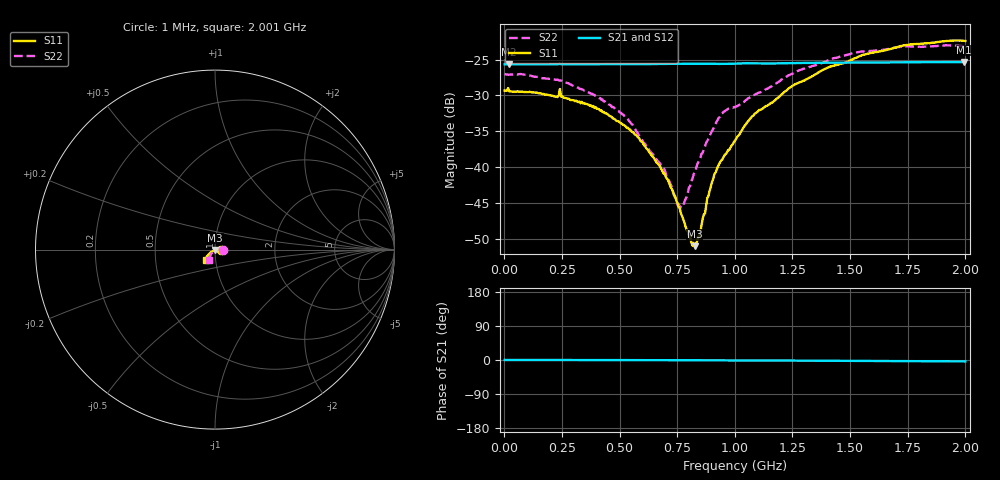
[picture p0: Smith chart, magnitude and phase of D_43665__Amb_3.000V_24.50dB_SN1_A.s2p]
! device id: 43665_
! dir: \\malibu\benchdata\1_engineers\tn_data\43665_75ohm\new\sparar\43665_\amb\3p000v\24p50db
! Serial: 1
! Insertion: A
! Temp: Amb
! VDD: 3.000V
! Attenuation Step: 24.50dB
! IDD: 1.450665e+00mA
! FILE NAME
! DATE 03-27-2009 08:39:23
! CORRECTED  DATA
#  Hz  S  RI  R  75
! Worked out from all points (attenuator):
!   401 points, 1 MHz to 2.001 GHz, reference 75 ohm
!   highest |S21| = -25.32 dB at 1.996 GHz (marker M1); lowest = -25.7 dB at 21 MHz (marker M2)
!   lowest |S11| = -51.0 dB at 826 MHz (marker M3), VSWR 1.01, Z = 75.1 - j0.413 ohm
!   |S11| at or under -10 dB: start of sweep to end of sweep
!   |S22| runs from -45.6 to -23.0 dB; largest |S21 - S12| = 0.00057
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1000000  0.0342 -0.000123  0.0522 3.89e-05  0.0521 -2.09e-05  0.0447 -0.000493
2.1e7  0.0338 0.000184  0.0521 -9.04e-06  0.0521 -2.11e-05  0.0442 0.000343
2.36e8  0.0316 0.00216  0.0523 -1.5e-05  0.0522 -2.33e-06  0.04 0.00545
3.36e8  0.0285 0.00246  0.0522 -0.000125  0.0522 -6.12e-05  0.0342 0.00668
5.26e8  0.0191 0.00234  0.0524 -0.000328  0.0524 -0.000243  0.0219 0.00438
6.71e8  0.0103 0.000319  0.0525 -0.000365  0.0525 -0.000263  0.0108 -0.000229
7.06e8  0.00832 -0.000264  0.0525 -0.000444  0.0526 -0.000303  0.0083 -0.00125
7.61e8  0.00493 -0.00156  0.0526 -0.000531  0.0527 -0.000407  0.00367 -0.00384
7.81e8  0.00365 -0.00191  0.0527 -0.000591  0.0527 -0.000447  0.00195 -0.00535
8.06e8  0.00217 -0.00243  0.0527 -0.000659  0.0527 -0.000547  -4.65e-05 -0.00738
8.26e8  0.000563 -0.00275  0.0527 -0.000719  0.0527 -0.000604  -0.00159 -0.00931
8.46e8  -0.000862 -0.00321  0.0527 -0.000786  0.0527 -0.000635  -0.00276 -0.0107
8.91e8  -0.00469 -0.00497  0.0527 -0.000948  0.0527 -0.000775  -0.00664 -0.0151
9.16e8  -0.00656 -0.00637  0.0526 -0.000991  0.0527 -0.00082  -0.00965 -0.0175
9.51e8  -0.00887 -0.0077  0.0526 -0.000941  0.0526 -0.000786  -0.0153 -0.0189
1.001e9  -0.0125 -0.00882  0.0527 -0.000822  0.0528 -0.000634  -0.0191 -0.0179
1.096e9  -0.0203 -0.0131  0.0529 -0.00133  0.053 -0.00114  -0.0218 -0.0242
1.336e9  -0.0348 -0.0254  0.0535 -0.00167  0.0536 -0.00144  -0.0299 -0.0411
1.511e9  -0.0437 -0.0357  0.0536 -0.00239  0.0538 -0.00214  -0.0341 -0.052
1.671e9  -0.0488 -0.0452  0.0537 -0.00278  0.0539 -0.00262  -0.0346 -0.0574
1.996e9  -0.0495 -0.0578  0.0541 -0.00349  0.0542 -0.0035  -0.032 -0.0607
2.001e9  -0.0494 -0.0577  0.054 -0.00352  0.0541 -0.00347  -0.0321 -0.0607
